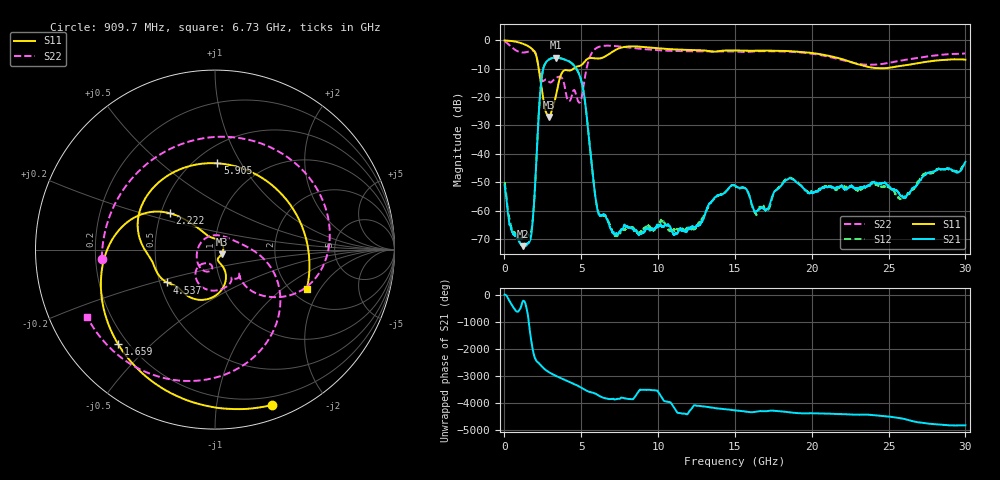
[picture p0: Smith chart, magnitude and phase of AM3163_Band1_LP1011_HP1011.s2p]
!Agilent Technologies,E8364B,MY43040894,A.07.50.67
!Agilent E8364B: A.07.50.67
!Date: Thursday, August 20, 2020 11:21:11
!Correction: S11(Full 2 Port(1,2))
!S21(Full 2 Port(1,2))
!S12(Full 2 Port(1,2))
!S22(Full 2 Port(1,2))
!S2P File: Measurements: S11, S21, S12, S22:
# Hz S  dB  R 50
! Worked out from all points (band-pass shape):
!   3201 points, 10 MHz to 30 GHz, reference 50 ohm
!   highest |S21| = -6.11 dB at 3.356 GHz (marker M1); lowest = -72.5 dB at 1.21 GHz (marker M2)
!   |S21| within 3 dB of the highest: 2.574 GHz to 4.562 GHz (1.988 GHz wide, 55.7 % of centre)
!   lowest |S11| = -27.0 dB at 2.906 GHz (marker M3), VSWR 1.09, Z = 53.7 - j2.72 ohm
!   |S11| at or under -10 dB: 2.226 GHz to 4.489 GHz (2.262 GHz wide, 67.4 % of centre)
!   |S22| runs from -22.0 to -0.4 dB; largest |S21 - S12| = 0.0032
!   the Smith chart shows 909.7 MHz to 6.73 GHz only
!   S11 on the Smith chart (normalised r, x): 909.7 MHz: 0.12, -1.43; 1.659 GHz: 0.16, -0.40; 2.222 GHz: 0.56, +0.25; 4.537 GHz: 0.55, -0.22; 5.905 GHz: 0.64, +0.80; 6.73 GHz: 2.41, -1.53
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1e7  -0.05 -5.0  -51.07 16.7  -49.99 19.6  -0.42 -16.1
4.129906e8  -0.21 -31.3  -66.01 55.8  -65.20 -42.5  -2.13 -89.2
9.097e8  -0.70 -69.8  -70.29 118.5  -69.32 -118.0  -3.98 -175.4
1.2096e9  -1.22 -94.3  -72.54 141.9  -69.33 62.8  -4.30 137.6
1.65945e9  -2.46 -135.9  -70.53 90.0  -68.99 -15.8  -3.80 65.1
2.221762e9  -9.84 141.2  -26.95 11.3  -26.88 11.0  -9.52 -46.8
2.905909e9  -27.03 -34.6  -6.72 25.2  -6.72 25.2  -14.66 -59.1
3.355759e9  -19.39 -65.1  -6.11 -109.6  -6.12 -109.6  -13.23 -74.7
3.964931e9  -10.47 -116.2  -6.87 98.4  -6.87 98.5  -17.58 -134.7
4.536616e9  -9.79 -145.6  -8.93 -45.6  -8.92 -45.6  -17.51 -120.9
5.014581e9  -8.69 -173.5  -14.54 171.3  -14.51 171.1  -20.47 45.6
5.904909e9  -6.36 88.3  -54.72 -38.9  -54.71 -39.5  -3.04 -87.2
6.729634e9  -5.09 -23.2  -63.81 122.4  -63.46 79.9  -1.88 -152.4
7.423153e9  -2.90 -100.4  -68.14 126.8  -68.55 104.5  -2.12 169.5
8.285366e9  -2.11 -168.7  -66.10 107.5  -65.96 112.1  -2.63 130.3
1.000979e10  -2.80 100.0  -65.68 15.6  -65.02 68.3  -3.50 62.5
1.22403e10  -3.43 10.6  -65.76 167.5  -66.42 -112.1  -3.87 -14.7
1.5005e10  -3.57 -71.5  -51.18 58.9  -51.28 59.1  -3.94 -93.1
2.000958e10  -4.45 163.2  -53.70 -47.0  -53.54 -47.9  -4.71 136.6
2.275554e10  -8.01 60.3  -52.13 -99.4  -52.12 -97.5  -8.00 21.0
2.500479e10  -9.70 -62.6  -51.37 -169.8  -51.73 -174.9  -7.97 -92.2
3e10  -6.82 104.4  -42.85 -134.1  -43.77 -137.5  -4.63 102.5
